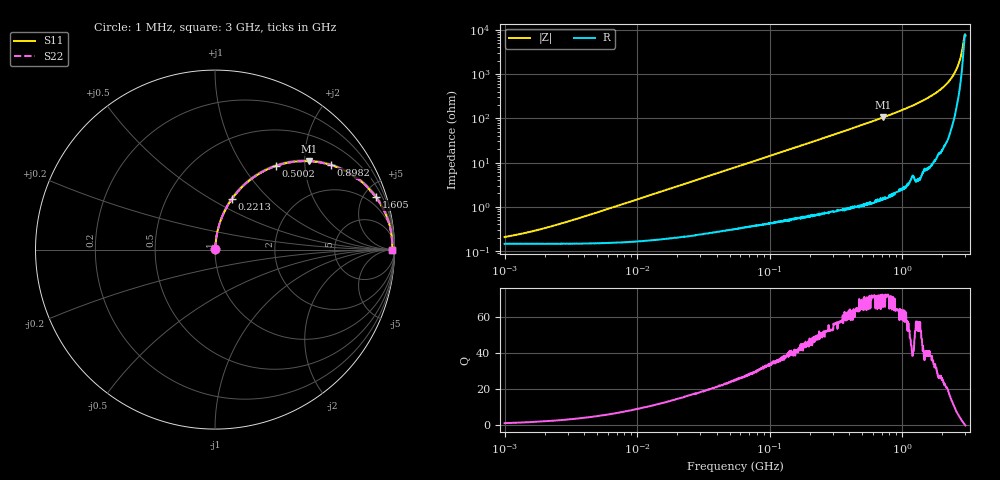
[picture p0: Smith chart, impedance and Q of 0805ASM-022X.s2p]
!s-Parameter Generated by FASTRON Sdn. Bhd.
!FASTRON P/N : 0805ASM-022X
!Keysight Technologies: E4991B_MY54100416_A.01.15
!Date: Fri Jun 19 14:48:00 2026
!Version  :Rev00  Fri Jun 19 14:48:00 2026
!Data & Calibration Information:
!Freq  S11  S21  S12  S22
!PortZ  Port1:50+j0  Port2:50+j0
!When reading reference impedance value at option line is always used.
! Remarks : This data is being provided solely for informational purposes.
# Hz S dB R 50
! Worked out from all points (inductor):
!   1601 points, 1 MHz to 3 GHz, reference 50 ohm
!   read as one part in series: L = 23.3 nH near 3.007 MHz
!   highest Q = 71.6 at 720.7 MHz (marker M1), where L = 23.2 nH
!   self-resonance near 2.97 GHz
!   S11 on the Smith chart (normalised r, x): 1 MHz: 1.00, +0.00; 221.3 MHz: 1.01, +0.62; 500.2 MHz: 1.02, +1.42; 898.2 MHz: 1.04, +2.70; 1.605 GHz: 1.16, +6.06; 3 GHz: open
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1000000  -53.70 45.3  -0.01 -0.1  -0.01 -0.1  -53.70 45.3
1822989  -50.30 61.3  -0.01 -0.2  -0.01 -0.2  -50.30 61.3
3804036  -44.80 74.9  -0.01 -0.3  -0.01 -0.3  -44.80 74.9
1.447069e7  -33.50 83.9  -0.02 -1.2  -0.02 -1.2  -33.50 83.9
5.504702e7  -22.20 83.3  -0.05 -4.5  -0.05 -4.5  -22.20 83.3
1.103592e8  -16.30 79.6  -0.14 -8.8  -0.14 -8.8  -16.30 79.6
2.083556e8  -11.10 72.6  -0.40 -16.1  -0.40 -16.1  -11.10 72.6
2.212502e8  -10.60 71.7  -0.45 -17.1  -0.45 -17.1  -10.60 71.7
3.368469e8  -7.45 63.9  -0.93 -25.1  -0.93 -25.1  -7.45 63.9
5.001674e8  -4.81 54.0  -1.83 -35.1  -1.83 -35.1  -4.81 54.0
7.207075e8  -2.86 43.2  -3.29 -46.0  -3.29 -46.0  -2.86 43.2
7.925923e8  -2.44 40.2  -3.81 -49.0  -3.81 -49.0  -2.44 40.2
8.982141e8  -1.96 36.2  -4.58 -52.9  -4.58 -52.9  -1.96 36.2
1.255985e9  -0.98 25.7  -7.26 -63.2  -7.26 -63.2  -0.98 25.7
1.604986e9  -0.51 18.1  -10.10 -70.4  -10.10 -70.4  -0.51 18.1
2.040726e9  -0.23 11.1  -14.30 -76.5  -14.30 -76.5  -0.23 11.1
2.244273e9  -0.16 8.3  -16.80 -78.5  -16.80 -78.5  -0.16 8.3
2.443543e9  -0.13 5.8  -19.80 -79.0  -19.80 -79.0  -0.13 5.8
2.687267e9  -0.11 3.1  -25.30 -75.3  -25.30 -75.3  -0.11 3.1
2.769173e9  -0.11 2.2  -28.00 -71.0  -28.00 -71.0  -0.11 2.2
2.911267e9  -0.11 0.7  -35.10 -44.7  -35.10 -44.7  -0.11 0.7
3e9  -0.11 -0.2  -37.70 15.4  -37.70 15.4  -0.11 -0.2
